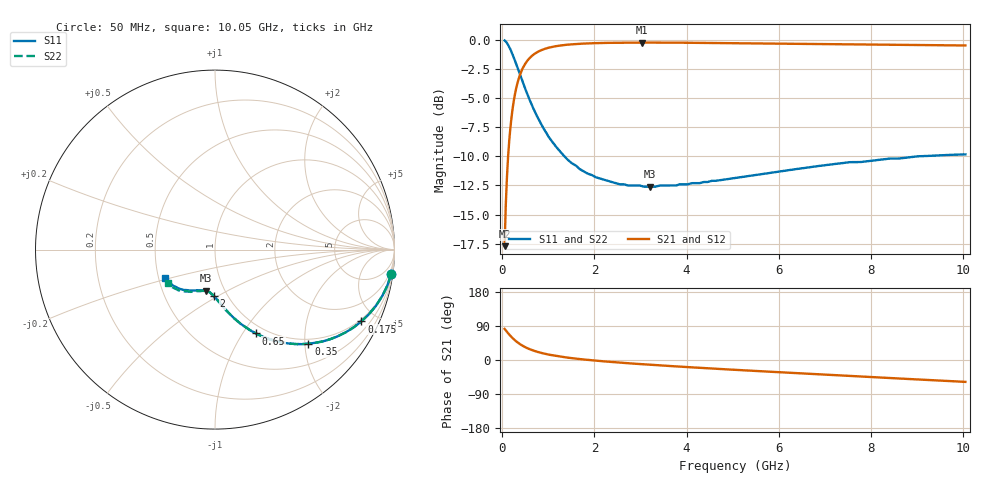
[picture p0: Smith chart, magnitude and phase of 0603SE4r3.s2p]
! AVX Thin Film Operation		Date: August 2001
! Description: Accu-P® Series, Thin Film, SMD, RF Capacitor
! Part Number: 06035J4R3ABT
! 50 MHz  -  10.05 GHz
! Serial Measurements
# mhz S db R 50
!	S11		S21		S12		S22
!	dB	Phase	dB	Phase	dB	Phase	dB	Phase
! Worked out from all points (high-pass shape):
!   401 points, 50 MHz to 10.05 GHz, reference 50 ohm
!   highest |S21| = -0.26 dB at 3.025 GHz (marker M1); lowest = -17.7 dB at 50 MHz (marker M2)
!   |S21| within 3 dB of the highest: 363.7 MHz to end of sweep
!   lowest |S11| = -12.6 dB at 3.2 GHz (marker M3), VSWR 1.61, Z = 40.9 - j19.8 ohm
!   |S11| at or under -10 dB: 1.347 GHz to 9.021 GHz (7.673 GHz wide, 148 % of centre)
!   |S22| runs from -12.5 to -0.1 dB; largest |S21 - S12| = 0
!   S11 on the Smith chart (normalised r, x): 50 MHz: 1, -14; 175 MHz: 0.90, -4.12; 350 MHz: 0.90, -2.08; 650 MHz: 0.90, -1.15; 2 GHz: 0.86, -0.48; 10.05 GHz: 0.54, -0.19
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50  -0.07 -7.9  -17.70 82.1  -17.70 82.1  -0.07 -7.9
75  -0.17 -11.8  -14.21 78.2  -14.21 78.2  -0.17 -11.8
125  -0.45 -19.3  -10.06 70.7  -10.06 70.7  -0.45 -19.3
175  -0.83 -26.1  -7.58 63.9  -7.58 63.9  -0.83 -26.1
250  -1.55 -35.3  -5.23 54.7  -5.23 54.7  -1.55 -35.3
350  -2.63 -45.2  -3.43 44.8  -3.43 44.8  -2.63 -45.2
425  -3.45 -51.2  -2.61 38.7  -2.61 38.7  -3.45 -51.2
500  -4.25 -56.2  -2.06 33.7  -2.06 33.7  -4.25 -56.2
650  -5.69 -64.0  -1.37 26.0  -1.37 26.0  -5.69 -64.0
825  -7.11 -70.6  -0.94 19.4  -0.94 19.4  -7.11 -70.5
1050  -8.56 -76.6  -0.66 13.3  -0.66 13.3  -8.55 -76.6
1400  -10.22 -83.5  -0.44 6.5  -0.44 6.5  -10.22 -83.3
1725  -11.20 -88.2  -0.35 1.9  -0.35 1.9  -11.20 -87.8
2000  -11.73 -91.5  -0.31 -1.4  -0.31 -1.4  -11.73 -91.1
2525  -12.37 -96.9  -0.27 -6.7  -0.27 -6.7  -12.37 -96.2
3025  -12.55 -101.5  -0.26 -11.1  -0.26 -11.1  -12.50 -100.5
3200  -12.60 -102.5  -0.26 -12.4  -0.26 -12.4  -12.50 -101.5
3400  -12.52 -104.8  -0.26 -14.0  -0.26 -14.0  -12.50 -103.0
5050  -11.86 -116.8  -0.31 -25.9  -0.31 -25.9  -11.86 -114.4
6725  -10.90 -128.0  -0.38 -36.8  -0.38 -36.8  -10.90 -125.0
8400  -10.20 -140.1  -0.46 -47.5  -0.46 -47.5  -10.19 -135.1
10050  -9.84 -150.6  -0.50 -57.7  -0.50 -57.7  -9.80 -144.6
